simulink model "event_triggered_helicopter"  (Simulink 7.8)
settings: Solver=ode45  StartTime=0.0  StopTime=89  RelTol=1e-3
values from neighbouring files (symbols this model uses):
  d = lambda*0.5    [main_epsilon.m]    (also in main_rho_tau.m = 0.5)
undefined symbols (not defined in the file or in its folder): Ac_epsilon, Ac_rho, Ac_tau, c_epsilon, DiscIntNeverNeededParam, epsilon_0, Epsilon_disc, g, J_epsilon, Ka, Kb, Kc, L_epsilon, L_rho, L_tau, la, lh, lw, m, M, M_bf, Rho_disc, Tau_disc
libraries: commnoisgen2 x6, dspswit3 x2

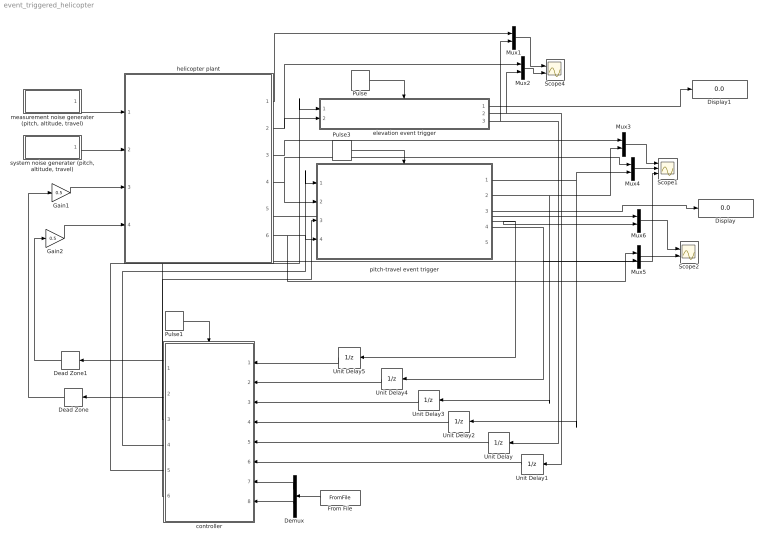
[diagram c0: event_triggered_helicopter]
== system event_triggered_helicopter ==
  Dead Zone : DeadZone  LowerValue=-1  UpperValue=1
  Dead Zone1 : DeadZone  LowerValue=-1  UpperValue=1
  Demux : Demux  Outputs=2
  Display : Display
  Display1 : Display
  From File : FromFile  FileName=input.mat  SampleTime=0
  Gain1 : Gain  Gain=0.5
  Gain2 : Gain  Gain=0.5
  Mux{1..6} (6 alike) : Mux  Inputs=2
  Pulse : DiscretePulseGenerator  PulseType=Time based  Period=0.005  PulseWidth=50
  Pulse1 : DiscretePulseGenerator  PulseType=Time based  Period=0.005  PulseWidth=30
  Pulse3 : DiscretePulseGenerator  PulseType=Time based  Period=0.005  PulseWidth=50
  Scope1 : Scope  NumInputPorts=3
  Scope2 : Scope  NumInputPorts=2
  Scope4 : Scope  NumInputPorts=2
  Unit Delay{,1..5} (6 alike) : UnitDelay  SampleTime=-1
  controller : Subsystem
  elevation event trigger : Subsystem
  helicopter plant : Subsystem
  "measurement noise generater (pitch, altitude, travel)" : Subsystem
  pitch-travel event trigger : Subsystem
  "system noise generater (pitch, altitude, travel)" : Subsystem
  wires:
  helicopter plant/2(altitude) -> elevation event trigger/2(elevation), Mux2/1
  Pulse/1 -> elevation event trigger/Trigger
  Mux1/1 -> Scope4/1
  Pulse1/1 -> controller/Trigger
  helicopter plant/5(travel rate) -> Mux6/1
  helicopter plant/3(pitch rate) -> Mux3/1
  controller/1(Vb) -> Dead Zone1/1
  Gain2/1 -> helicopter plant/4(Tb)
  controller/2(Vf) -> Dead Zone/1
  Gain1/1 -> helicopter plant/3(Tf)
  controller/5(u_elv) -> elevation event trigger/1(u_elv)
  From File/1 -> Demux/1
  Demux/2 -> controller/8(travel_rate_offset)
  Demux/1 -> controller/7(elevation_offset)
  helicopter plant/1(altitude rate) -> Mux1/1
  Mux2/1 -> Scope4/2
  elevation event trigger/3(remote estimated elevation rate) -> Unit Delay/1, Mux1/2
  elevation event trigger/2(remote estimated elevation) -> Unit Delay1/1, Mux2/2
  Unit Delay/1 -> controller/5(elevation_rate)
  Unit Delay1/1 -> controller/6(elevation)
  helicopter plant/4(pitch) -> pitch-travel event trigger/2(pitch), Mux4/1
  Unit Delay2/1 -> controller/4(pitch)
  Mux3/1 -> Scope1/1
  Mux4/1 -> Scope1/2
  Pulse3/1 -> pitch-travel event trigger/Trigger
  helicopter plant/6(travel) -> pitch-travel event trigger/4(travel), Mux5/1
  controller/3(u_trv) -> pitch-travel event trigger/3(u_trv)
  controller/4(u_pth) -> pitch-travel event trigger/1(u_pth)
  Mux5/1 -> Scope2/2
  pitch-travel event trigger/4("remote estimated travel ") -> Unit Delay4/1, Mux5/2
  Unit Delay3/1 -> controller/3(pitch_rate)
  Unit Delay4/1 -> controller/2(travel)
  pitch-travel event trigger/5(remote estimated travel rate) -> Mux6/2, Unit Delay5/1
  Mux6/1 -> Scope2/1
  Unit Delay5/1 -> controller/1(travel_rate)
  "measurement noise generater (pitch, altitude, travel)"/1(measurement noise) -> helicopter plant/1("measurement noise (pitch, altitude, travel)")
  "system noise generater (pitch, altitude, travel)"/1(system noise) -> helicopter plant/2("system noise (pitch, altitude, travel)")
  Dead Zone/1 -> Gain1/1
  Dead Zone1/1 -> Gain2/1
  pitch-travel event trigger/1(remote estimated pitch) -> Mux4/2, Unit Delay2/1
  pitch-travel event trigger/2(remote estimated pitch rate) -> Mux3/2, Unit Delay3/1
  pitch-travel event trigger/3(transmission times) -> Display/1
  elevation event trigger/1(elevation transmission times) -> Display1/1
  controller/6(pitch_offset) -> Scope1/3

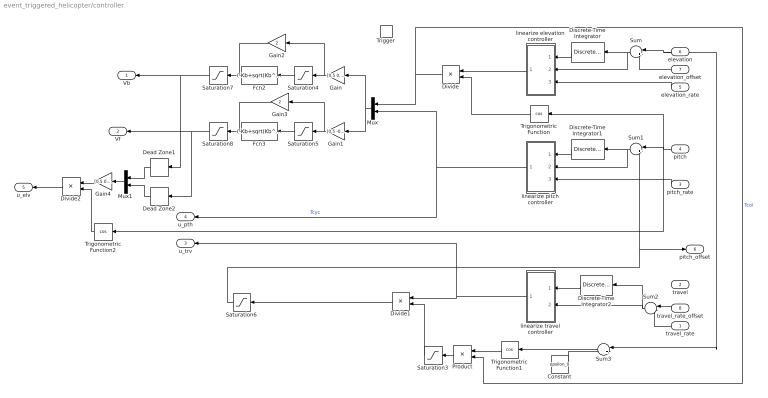
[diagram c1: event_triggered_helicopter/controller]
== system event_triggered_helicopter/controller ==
  travel_rate : Inport
  travel : Inport  Port=2
  pitch_rate : Inport  Port=3
  pitch : Inport  Port=4
  elevation_rate : Inport  Port=5
  elevation : Inport  Port=6
  elevation_offset : Inport  Port=7
  travel_rate_offset : Inport  Port=8
  Trigger : TriggerPort
  Constant : Constant  Value=epsilon_0
  Dead Zone1 : DeadZone  LowerValue=-1  UpperValue=1
  Dead Zone2 : DeadZone  LowerValue=-1  UpperValue=1
  Discrete-Time Integrator : DiscreteIntegrator  SampleTime=-1  LimitOutput=on  UpperSaturationLimit=1.8  LowerSaturationLimit=-1.8  ICPrevOutput=DiscIntNeverNeededParam  ICPrevScaledInput=DiscIntNeverNeededParam
  Discrete-Time Integrator1 : DiscreteIntegrator  SampleTime=-1  LimitOutput=on  UpperSaturationLimit=0.5  LowerSaturationLimit=-0.5  ICPrevOutput=DiscIntNeverNeededParam  ICPrevScaledInput=DiscIntNeverNeededParam
  Discrete-Time Integrator2 : DiscreteIntegrator  SampleTime=-1  LimitOutput=on  UpperSaturationLimit=0.12  LowerSaturationLimit=-0.12  ICPrevOutput=DiscIntNeverNeededParam  ICPrevScaledInput=DiscIntNeverNeededParam
  Divide : Product  Inputs=*/
  Divide1 : Product  Inputs=*/
  Divide2 : Product  Inputs=**
  Fcn2 : Fcn  Expr=(-Kb+sqrt(Kb^2-4*Ka*(Kc-u(1))))/(2*Ka)
  Fcn3 : Fcn  Expr=(-Kb+sqrt(Kb^2-4*Ka*(Kc-u(1))))/(2*Ka)
  Gain : Gain  Gain=[0.5 0.5]  Multiplication=Matrix(K*u)
  Gain1 : Gain  Gain=[0.5 -0.5]  Multiplication=Matrix(K*u)
  Gain2 : Gain  Gain=2
  Gain3 : Gain  Gain=2
  Gain4 : Gain  Gain=[0.5 0.5]  Multiplication=Matrix(K*u)
  Mux : Mux  Inputs=2
  Mux1 : Mux  Inputs=2
  Product : Product
  Saturation3 : Saturate  UpperLimit=inf  LowerLimit=0.8
  Saturation4 : Saturate  UpperLimit=1  LowerLimit=-0.0012
  Saturation5 : Saturate  UpperLimit=1  LowerLimit=-0.0012
  Saturation6 : Saturate  UpperLimit=0.6  LowerLimit=-0.6
  Saturation7 : Saturate  UpperLimit=4.99  LowerLimit=-4.99
  Saturation8 : Saturate  UpperLimit=4.99  LowerLimit=-4.99
  Sum : Sum  Inputs=|+-
  Sum1 : Sum  Inputs=|+-
  Sum2 : Sum  Inputs=|-+
  Sum3 : Sum  Inputs=|+-
  Trigonometric Function : Trigonometry  Operator=cos
  Trigonometric Function1 : Trigonometry  Operator=cos
  Trigonometric Function2 : Trigonometry  Operator=cos
  linearize elevation controller : Subsystem
  linearize pitch controller : Subsystem
  linearize travel controller : Subsystem
  Vb : Outport
  Vf : Outport  Port=2
  u_trv : Outport  Port=3
  u_pth : Outport  Port=4
  u_elv : Outport  Port=5
  pitch_offset : Outport  Port=6
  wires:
  elevation/1 -> Sum/1, Sum3/1
  elevation_offset/1 -> Sum/2
  Sum/1 -> linearize elevation controller/2(P), Discrete-Time Integrator/1
  Discrete-Time Integrator/1 -> linearize elevation controller/1(I)
  elevation_rate/1 -> linearize elevation controller/3(D)
  pitch/1 -> Sum1/1, Trigonometric Function2/1, Trigonometric Function/1
  Sum1/1 -> linearize pitch controller/2(P), Discrete-Time Integrator1/1
  pitch_rate/1 -> linearize pitch controller/3(D)
  travel_rate_offset/1 -> Sum2/1
  travel_rate/1 -> Sum2/2
  Sum2/1 -> Discrete-Time Integrator2/1, linearize travel controller/2(P)
  Discrete-Time Integrator2/1 -> linearize travel controller/1(I)
  Sum3/1 -> Trigonometric Function1/1
  Trigonometric Function1/1 -> Product/1
  Divide/1 -> Mux/1, Product/2  "Tcol"
  Product/1 -> Saturation3/1
  Saturation3/1 -> Divide1/2
  Mux/1 -> Gain/1, Gain1/1
  Gain/1 -> Saturation4/1, Gain2/1
  Gain1/1 -> Saturation5/1, Gain3/1
  Divide1/1 -> Saturation6/1
  Saturation7/1 -> Vb/1, Dead Zone1/1
  Saturation8/1 -> Vf/1, Dead Zone2/1
  Constant/1 -> Sum3/2
  Saturation4/1 -> Fcn2/1
  Saturation5/1 -> Fcn3/1
  Trigonometric Function/1 -> Divide/2
  Discrete-Time Integrator1/1 -> linearize pitch controller/1(I)
  Gain2/1 -> Saturation7/1
  Gain3/1 -> Saturation8/1
  linearize pitch controller/1(u_pth) -> Mux/2, u_pth/1  "Tcyc"
  linearize travel controller/1(u_trv) -> Divide1/1, u_trv/1
  linearize elevation controller/1(u_elv) -> Divide/1
  Dead Zone1/1 -> Mux1/1
  Dead Zone2/1 -> Mux1/2
  Mux1/1 -> Gain4/1
  Gain4/1 -> Divide2/1
  Trigonometric Function2/1 -> Divide2/2
  Divide2/1 -> u_elv/1
  Saturation6/1 -> Sum1/2, pitch_offset/1

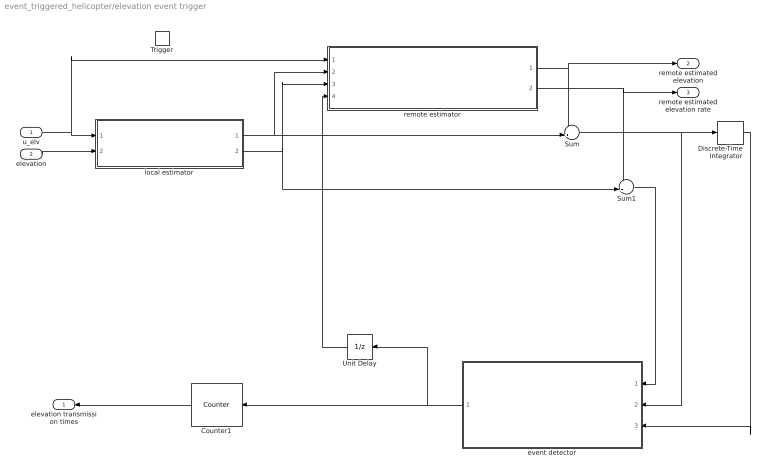
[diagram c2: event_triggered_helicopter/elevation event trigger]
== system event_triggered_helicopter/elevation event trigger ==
  u_elv : Inport
  elevation : Inport  Port=2
  Trigger : TriggerPort
  Counter1 : dspswit3/Counter  Direction=Up  CountEvent=Non-zero sample  CounterSize=User defined  MaxCount=20000  InitialCount=0  Output=Count  HitValue=32  ResetInput=off  SamplesPerFrame=1  Ts=1  CntDtype=int32  HitDtype=Logical
  Discrete-Time Integrator : DiscreteIntegrator  SampleTime=-1  ICPrevOutput=DiscIntNeverNeededParam  ICPrevScaledInput=DiscIntNeverNeededParam
  Sum : Sum  Inputs=-+|
  Sum1 : Sum  Inputs=-+|
  Unit Delay : UnitDelay  SampleTime=-1
  event detector : Subsystem
  local estimator : Subsystem
  remote estimator : Subsystem
  elevation transmission times : Outport
  remote estimated elevation : Outport  Port=2
  remote estimated elevation rate : Outport  Port=3
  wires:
  u_elv/1 -> local estimator/1(u_elv), remote estimator/1(u_elv)
  elevation/1 -> local estimator/2(elevation)
  local estimator/1(local estimated elevation) -> remote estimator/2("local estimated elevation "), Sum/2
  remote estimator/1(remote estimated elevation) -> remote estimated elevation/1, Sum/1
  local estimator/2(local estimated elevation rate) -> remote estimator/3(local estimated elevation rate), Sum1/2
  Counter1/1 -> elevation transmission times/1
  Unit Delay/1 -> remote estimator/4(transmit signal)
  remote estimator/2(remote estimated elevation rate) -> remote estimated elevation rate/1, Sum1/1
  event detector/1(transmit signal) -> Unit Delay/1, Counter1/1
  Sum/1 -> Discrete-Time Integrator/1, event detector/2(elevation_p)
  Sum1/1 -> event detector/1(elevation_d)
  Discrete-Time Integrator/1 -> event detector/3(elevation_i)

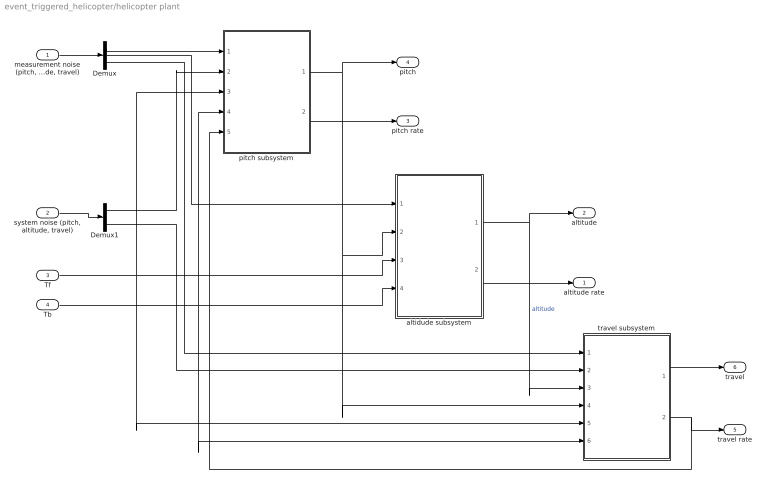
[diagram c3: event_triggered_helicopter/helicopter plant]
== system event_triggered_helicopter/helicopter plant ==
  "measurement noise (pitch, altitude, travel)" : Inport
  "system noise (pitch, altitude, travel)" : Inport  Port=2
  Tf : Inport  Port=3
  Tb : Inport  Port=4
  Demux : Demux  Outputs=3
  Demux1 : Demux  Outputs=3
  altidude subsystem : Subsystem
  pitch subsystem : Subsystem
  travel subsystem : Subsystem
  altitude rate : Outport
  altitude : Outport  Port=2
  pitch rate : Outport  Port=3
  pitch : Outport  Port=4
  travel rate : Outport  Port=5
  travel : Outport  Port=6
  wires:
  pitch subsystem/1(pitch) -> pitch/1, altidude subsystem/2(pitch), travel subsystem/4(pitch)
  altidude subsystem/1(altitude) -> altitude/1, travel subsystem/3(altitude)  "altitude"
  pitch subsystem/2(pitch rate) -> pitch rate/1
  altidude subsystem/2(altitude rate) -> altitude rate/1
  travel subsystem/1(travel) -> travel/1
  travel subsystem/2(travel rate) -> pitch subsystem/5(travel_rate), travel rate/1
  Demux/1 -> pitch subsystem/1(measurement noise)
  Demux/2 -> altidude subsystem/1(measurement noise)
  Demux/3 -> travel subsystem/1(measurement noise)
  "measurement noise (pitch, altitude, travel)"/1 -> Demux/1
  Demux1/1 -> pitch subsystem/2(system noise)
  Demux1/3 -> travel subsystem/2(system noise)
  Tf/1 -> altidude subsystem/3(Tf), travel subsystem/5(Tf), pitch subsystem/3(Tf)
  Tb/1 -> altidude subsystem/4(Tb), pitch subsystem/4(Tb), travel subsystem/6(Tb)
  "system noise (pitch, altitude, travel)"/1 -> Demux1/1

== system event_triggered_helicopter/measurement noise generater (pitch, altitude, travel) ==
  Mux : Mux  Inputs=3
  altitude Noise Generator : commnoisgen2/Gaussian Noise Generator  m=0  d=1.857e-8  s=41  Ts=0.0025  frameBased=off  sampPerFrame=1  orient=off  outDataType=double
  pitch noise Generator : commnoisgen2/Gaussian Noise Generator  m=0  d=1.857e-8  s=1  Ts=0.0025  frameBased=off  sampPerFrame=1  orient=off  outDataType=double
  travel noise Generator : commnoisgen2/Gaussian Noise Generator  m=0  d=1.857e-8  s=3  Ts=0.0025  frameBased=off  sampPerFrame=1  orient=off  outDataType=double
  measurement noise : Outport
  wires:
  pitch noise Generator/1 -> Mux/1
  altitude Noise Generator/1 -> Mux/2
  travel noise Generator/1 -> Mux/3
  Mux/1 -> measurement noise/1

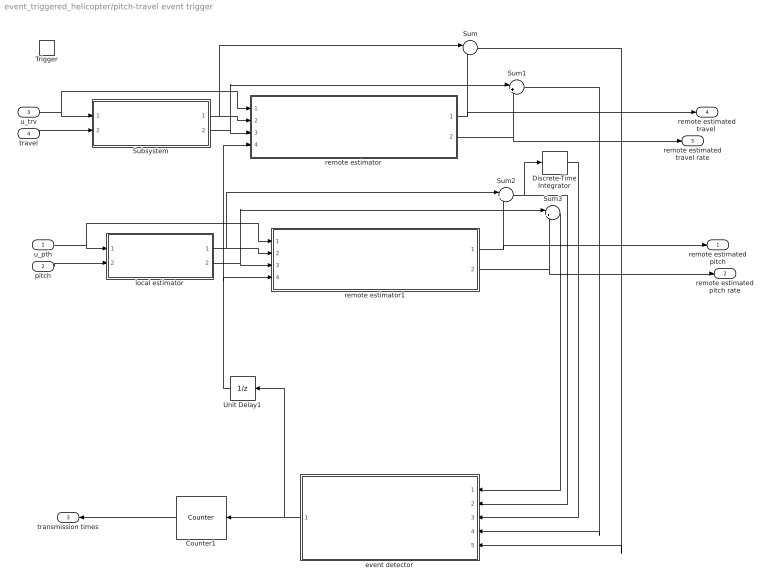
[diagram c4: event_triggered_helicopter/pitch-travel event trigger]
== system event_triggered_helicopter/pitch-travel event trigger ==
  u_pth : Inport
  pitch : Inport  Port=2
  u_trv : Inport  Port=3
  travel : Inport  Port=4
  Trigger : TriggerPort
  Counter1 : dspswit3/Counter  Direction=Up  CountEvent=Non-zero sample  CounterSize=User defined  MaxCount=20000  InitialCount=0  Output=Count  HitValue=32  ResetInput=off  SamplesPerFrame=1  Ts=1  CntDtype=int32  HitDtype=Logical
  Discrete-Time Integrator : DiscreteIntegrator  SampleTime=-1  ICPrevOutput=DiscIntNeverNeededParam  ICPrevScaledInput=DiscIntNeverNeededParam
  Subsystem : Subsystem
  Sum{,1..3} (4 alike) : Sum  Inputs=|+-
  Unit Delay1 : UnitDelay  SampleTime=-1
  event detector : Subsystem
  local estimator : Subsystem
  remote estimator : Subsystem
  remote estimator1 : Subsystem
  remote estimated pitch : Outport
  remote estimated pitch rate : Outport  Port=2
  transmission times : Outport  Port=3
  "remote estimated travel " : Outport  Port=4
  remote estimated travel rate : Outport  Port=5
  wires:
  u_trv/1 -> Subsystem/1(u_trv), remote estimator/1(u_trv)
  travel/1 -> Subsystem/2(travel)
  Subsystem/2(local estimated travel rate) -> remote estimator/3(local estimated travel rate), Sum1/1
  remote estimator/2(remote estimated travel rate) -> remote estimated travel rate/1, Sum1/2
  remote estimator/1(remote estimated travel) -> "remote estimated travel "/1, Sum/2
  Subsystem/1(local estimated travel) -> remote estimator/2(local estimated travel), Sum/1
  Counter1/1 -> transmission times/1
  event detector/1(transmit signal) -> Unit Delay1/1, Counter1/1
  u_pth/1 -> local estimator/1(u_pth), remote estimator1/1(u_pth)
  pitch/1 -> local estimator/2(pitch)
  local estimator/1(local estimated pitch) -> remote estimator1/2(local estimated pitch), Sum2/1
  local estimator/2(local estimated pitch rate) -> remote estimator1/3(local estimated pitch rate), Sum3/1
  remote estimator1/1(remote estimated pitch) -> remote estimated pitch/1, Sum2/2
  remote estimator1/2(remote estimated pitch rate) -> remote estimated pitch rate/1, Sum3/2
  Sum2/1 -> Discrete-Time Integrator/1, event detector/2(pitch_p)
  Sum3/1 -> event detector/1(pitch_d)
  Discrete-Time Integrator/1 -> event detector/3(pitch_i)
  Sum1/1 -> event detector/4(travel_d)
  Sum/1 -> event detector/5(travel_p)
  Unit Delay1/1 -> remote estimator/4(transmit signal), remote estimator1/4(transmit signal)

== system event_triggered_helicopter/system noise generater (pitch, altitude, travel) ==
  Mux : Mux  Inputs=3
  altitude Noise Generator : commnoisgen2/Gaussian Noise Generator  m=0  d=1e-12  s=7  Ts=0.0025  frameBased=off  sampPerFrame=1  orient=off  outDataType=double
  pitch noise Generator : commnoisgen2/Gaussian Noise Generator  m=0  d=1e-12  s=5  Ts=0.0025  frameBased=off  sampPerFrame=1  orient=off  outDataType=double
  travel Noise Generator : commnoisgen2/Gaussian Noise Generator  m=0  d=1e-12  s=11  Ts=0.0025  frameBased=off  sampPerFrame=1  orient=off  outDataType=double
  system noise : Outport
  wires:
  pitch noise Generator/1 -> Mux/1
  altitude Noise Generator/1 -> Mux/2
  Mux/1 -> system noise/1
  travel Noise Generator/1 -> Mux/3

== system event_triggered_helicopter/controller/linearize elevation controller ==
  I : Inport
  P : Inport  Port=2
  D : Inport  Port=3
  Gain : Gain  Gain=[-7 -44 -68]  Multiplication=Matrix(K*u)
  Mux : Mux  Inputs=3
  u_elv : Outport
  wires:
  Mux/1 -> Gain/1
  I/1 -> Mux/1
  Gain/1 -> u_elv/1
  P/1 -> Mux/2
  D/1 -> Mux/3

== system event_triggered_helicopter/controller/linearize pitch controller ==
  I : Inport
  P : Inport  Port=2
  D : Inport  Port=3
  Gain : Gain  Gain=[-3.5 -30 -20]  Multiplication=Matrix(K*u)
  Mux : Mux  Inputs=3
  u_pth : Outport
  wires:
  Mux/1 -> Gain/1
  I/1 -> Mux/1
  Gain/1 -> u_pth/1
  P/1 -> Mux/2
  D/1 -> Mux/3

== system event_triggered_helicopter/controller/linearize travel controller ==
  I : Inport
  P : Inport  Port=2
  Gain : Gain  Gain=[3.5 20]  Multiplication=Matrix(K*u)
  Mux : Mux  Inputs=2
  u_trv : Outport
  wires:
  Mux/1 -> Gain/1
  I/1 -> Mux/1
  Gain/1 -> u_trv/1
  P/1 -> Mux/2

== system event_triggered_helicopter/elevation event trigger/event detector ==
  elevation_d : Inport
  elevation_p : Inport  Port=2
  elevation_i : Inport  Port=3
  Constant : Constant
  Constant1 : Constant  Value=0
  Fcn : Fcn  Expr=|
      | 7.5776*u(1)^6 + 0.064983*u(1)^5*u(2) + 0.0017543*u(1)^5*u(3) - 3.0262*u(1)^4*u(2)^2 
      |   - 0.0045238*u(1)^4*u(2)*u(3) + 3.6614*u(1)^4*u(3)^2 - 4.7737*u(1)^4 - 0.023298
      |   *u(1)^3*u(2)^3 - 0.001249*u(1)^3*u(2)^2*u(3) - 0.010189*u(1)^3*u(2)*u(3)^2 - 0.32359
      |   *u(1)^3*u(2) + 0.00012009*u(1)^3*u(3)^3 - 0.0078634*u(1)^3*u(3) + 1.106*u(1)^2*u(2)^4 
      |   + 0.0035527*u(1)^2*u(2)^3*u(3) - 0.99402*u(1)^2*u(2)^2*u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
  Mux : Mux  Inputs=3
  Switch : Switch
  transmit signal : Outport
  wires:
  elevation_d/1 -> Mux/3
  elevation_p/1 -> Mux/2
  elevation_i/1 -> Mux/1
  Mux/1 -> Fcn/1
  Fcn/1 -> Switch/2
  Constant/1 -> Switch/1
  Constant1/1 -> Switch/3
  Switch/1 -> transmit signal/1

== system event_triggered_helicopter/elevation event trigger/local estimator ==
  u_elv : Inport
  elevation : Inport  Port=2
  Demux : Demux  Outputs=2
  Gain2 : Gain  Gain=[Ac_epsilon(2:3,2:3) Epsilon_disc.B(2:3) L_epsilon(2:3,2)]  Multiplication=Matrix(K*u)
  Mux : Mux  Inputs=3
  Unit Delay : UnitDelay  SampleTime=-1
  local estimated elevation : Outport
  local estimated elevation rate : Outport  Port=2
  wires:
  Unit Delay/1 -> Mux/1
  u_elv/1 -> Mux/2
  elevation/1 -> Mux/3
  Mux/1 -> Gain2/1
  Gain2/1 -> Demux/1, Unit Delay/1
  Demux/1 -> local estimated elevation/1
  Demux/2 -> local estimated elevation rate/1

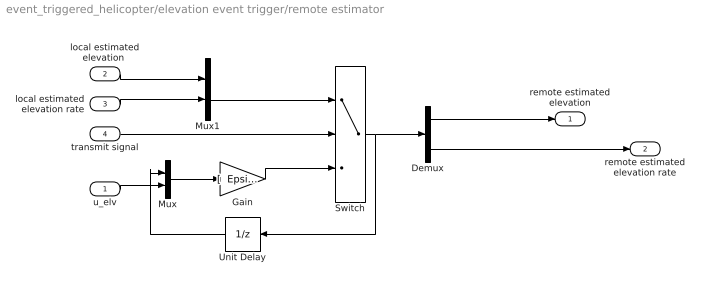
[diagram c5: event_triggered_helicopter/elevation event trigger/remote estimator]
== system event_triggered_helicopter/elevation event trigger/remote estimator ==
  u_elv : Inport
  "local estimated elevation " : Inport  Port=2
  local estimated elevation rate : Inport  Port=3
  transmit signal : Inport  Port=4
  Demux : Demux  Outputs=2
  Gain : Gain  Gain="[  Epsilon_disc.A(2:3,2:3)  Epsilon_disc.B(2:3)]"  Multiplication=Matrix(K*u)
  Mux : Mux  Inputs=2
  Mux1 : Mux  Inputs=2
  Switch : Switch  Threshold=1
  Unit Delay : UnitDelay  SampleTime=-1
  remote estimated elevation : Outport
  remote estimated elevation rate : Outport  Port=2
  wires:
  Mux/1 -> Gain/1
  u_elv/1 -> Mux/2
  Demux/1 -> remote estimated elevation/1
  Demux/2 -> remote estimated elevation rate/1
  Gain/1 -> Switch/3
  transmit signal/1 -> Switch/2
  Switch/1 -> Demux/1, Unit Delay/1
  Unit Delay/1 -> Mux/1
  "local estimated elevation "/1 -> Mux1/1
  local estimated elevation rate/1 -> Mux1/2
  Mux1/1 -> Switch/1

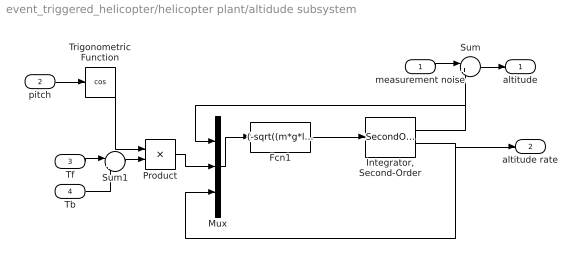
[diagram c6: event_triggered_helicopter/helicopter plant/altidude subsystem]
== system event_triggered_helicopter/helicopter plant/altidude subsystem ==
  measurement noise : Inport
  pitch : Inport  Port=2
  Tf : Inport  Port=3
  Tb : Inport  Port=4
  Fcn1 : Fcn  Expr=(-sqrt((m*g*lw-M*g*la)^2+((m+M)*g*d)^2)*sin(u(1))+(la+d*tan(u(1)+epsilon_0))*u(2)-c_epsilon*u(3))/J_epsilon
  "Integrator, Second-Order" : SecondOrderIntegrator
  Mux : Mux  Inputs=3
  Product : Product
  Sum : Sum  Inputs=|++
  Sum1 : Sum  Inputs=|++
  Trigonometric Function : Trigonometry  Operator=cos
  altitude : Outport
  altitude rate : Outport  Port=2
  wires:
  Fcn1/1 -> "Integrator, Second-Order"/1
  "Integrator, Second-Order"/1 -> Sum/2, Mux/1
  measurement noise/1 -> Sum/1
  Sum/1 -> altitude/1
  "Integrator, Second-Order"/2 -> altitude rate/1, Mux/3
  Tf/1 -> Sum1/1
  Tb/1 -> Sum1/2
  Mux/1 -> Fcn1/1
  Sum1/1 -> Product/2
  pitch/1 -> Trigonometric Function/1
  Product/1 -> Mux/2
  Trigonometric Function/1 -> Product/1

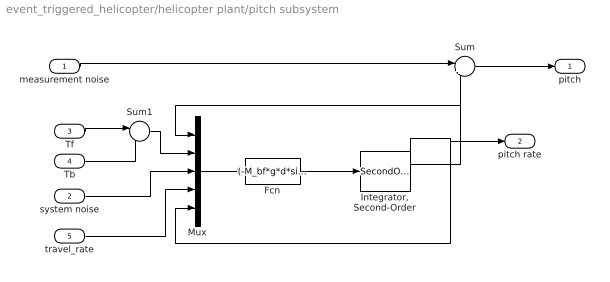
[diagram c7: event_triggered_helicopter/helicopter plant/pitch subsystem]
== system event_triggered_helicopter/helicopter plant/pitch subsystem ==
  measurement noise : Inport
  system noise : Inport  Port=2
  Tf : Inport  Port=3
  Tb : Inport  Port=4
  travel_rate : Inport  Port=5
  Fcn : Fcn  Expr=(-M_bf*g*d*sin(u(1))+lh*u(2)-0.003*u(5)+0.003*u(4)+u(3))/(0.01)
  "Integrator, Second-Order" : SecondOrderIntegrator
  Mux : Mux  Inputs=5
  Sum : Sum  Inputs=|++
  Sum1 : Sum  Inputs=|-+
  pitch : Outport
  pitch rate : Outport  Port=2
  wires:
  Mux/1 -> Fcn/1
  Fcn/1 -> "Integrator, Second-Order"/1
  "Integrator, Second-Order"/1 -> Sum/2, Mux/1
  measurement noise/1 -> Sum/1
  Sum/1 -> pitch/1
  "Integrator, Second-Order"/2 -> pitch rate/1, Mux/5
  system noise/1 -> Mux/3
  Tf/1 -> Sum1/1
  Tb/1 -> Sum1/2
  travel_rate/1 -> Mux/4
  Sum1/1 -> Mux/2

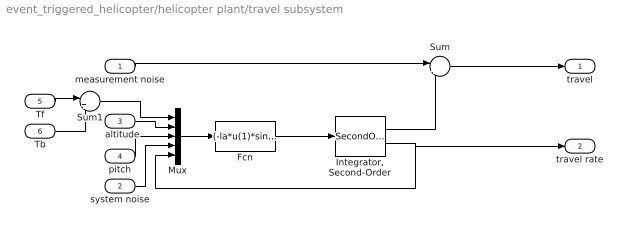
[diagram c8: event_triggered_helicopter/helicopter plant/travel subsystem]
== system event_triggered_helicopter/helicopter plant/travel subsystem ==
  measurement noise : Inport
  system noise : Inport  Port=2
  altitude : Inport  Port=3
  pitch : Inport  Port=4
  Tf : Inport  Port=5
  Tb : Inport  Port=6
  Fcn : Fcn  Expr=(-la*u(1)*sin(u(3))*cos(u(2)+epsilon_0)-0.25*u(5)+u(4))/4
  "Integrator, Second-Order" : SecondOrderIntegrator
  Mux : Mux  Inputs=5
  Sum : Sum  Inputs=|++
  Sum1 : Sum  Inputs=|++
  travel : Outport
  travel rate : Outport  Port=2
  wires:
  Mux/1 -> Fcn/1
  "Integrator, Second-Order"/1 -> Sum/2
  measurement noise/1 -> Sum/1
  Sum/1 -> travel/1
  altitude/1 -> Mux/2
  "Integrator, Second-Order"/2 -> travel rate/1, Mux/5
  Sum1/1 -> Mux/1
  pitch/1 -> Mux/3
  system noise/1 -> Mux/4
  Tf/1 -> Sum1/1
  Tb/1 -> Sum1/2
  Fcn/1 -> "Integrator, Second-Order"/1

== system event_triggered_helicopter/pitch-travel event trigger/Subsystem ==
  u_trv : Inport
  travel : Inport  Port=2
  Demux : Demux  Outputs=2
  Gain2 : Gain  Gain=[Ac_tau Tau_disc.B L_tau]  Multiplication=Matrix(K*u)
  Mux : Mux  Inputs=3
  Unit Delay : UnitDelay  SampleTime=-1
  local estimated travel : Outport
  local estimated travel rate : Outport  Port=2
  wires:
  Gain2/1 -> Unit Delay/1, Demux/1
  Unit Delay/1 -> Mux/1
  Mux/1 -> Gain2/1
  u_trv/1 -> Mux/2
  travel/1 -> Mux/3
  Demux/1 -> local estimated travel/1
  Demux/2 -> local estimated travel rate/1

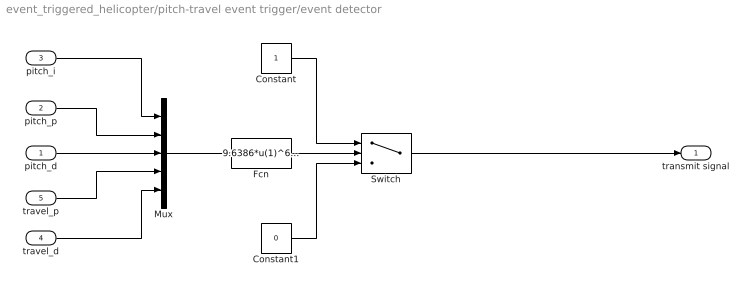
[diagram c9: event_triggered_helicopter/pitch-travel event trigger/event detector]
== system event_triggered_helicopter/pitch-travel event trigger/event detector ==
  pitch_d : Inport
  pitch_p : Inport  Port=2
  pitch_i : Inport  Port=3
  travel_d : Inport  Port=4
  travel_p : Inport  Port=5
  Constant : Constant
  Constant1 : Constant  Value=0
  Fcn : Fcn  Expr=|
      | 9.6386*u(1)^6 + 0.12666*u(1)^5*u(2) + 0.042053*u(1)^5*u(3) - 2.5554*u(1)^4*u(2)^2 + 0.33103
      |   *u(1)^4*u(2)*u(3) + 7.9379*u(1)^4*u(3)^2 - 10.9657*u(1)^4 - 0.064688*u(1)^3*u(2)^3 - 0.021023
      |   *u(1)^3*u(2)^2*u(3) + 0.024183*u(1)^3*u(2)*u(3)^2 - 0.22301*u(1)^3*u(2) + 0.0071206*u(1)^3
      |   *u(3)^3 - 0.031978*u(1)^3*u(3) + 2.0293*u(1)^2*u(2)^4 - 0.25656*u(1)^2*u(2)^3*u(3) - 1.2305
      |   *u(1)^2*u(2)^2*u(3)^2 +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
  Mux : Mux  Inputs=5
  Switch : Switch
  transmit signal : Outport
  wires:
  pitch_d/1 -> Mux/3
  pitch_p/1 -> Mux/2
  pitch_i/1 -> Mux/1
  travel_p/1 -> Mux/4
  travel_d/1 -> Mux/5
  Mux/1 -> Fcn/1
  Fcn/1 -> Switch/2
  Constant/1 -> Switch/1
  Constant1/1 -> Switch/3
  Switch/1 -> transmit signal/1

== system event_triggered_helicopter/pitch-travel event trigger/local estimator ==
  u_pth : Inport
  pitch : Inport  Port=2
  Demux : Demux  Outputs=2
  Gain2 : Gain  Gain=[Ac_rho(2:3,2:3) Rho_disc.B(2:3) L_rho(2:3,2)]  Multiplication=Matrix(K*u)
  Mux : Mux  Inputs=3
  Unit Delay : UnitDelay  SampleTime=-1
  local estimated pitch : Outport
  local estimated pitch rate : Outport  Port=2
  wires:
  Gain2/1 -> Unit Delay/1, Demux/1
  Unit Delay/1 -> Mux/1
  Mux/1 -> Gain2/1
  u_pth/1 -> Mux/2
  pitch/1 -> Mux/3
  Demux/1 -> local estimated pitch/1
  Demux/2 -> local estimated pitch rate/1

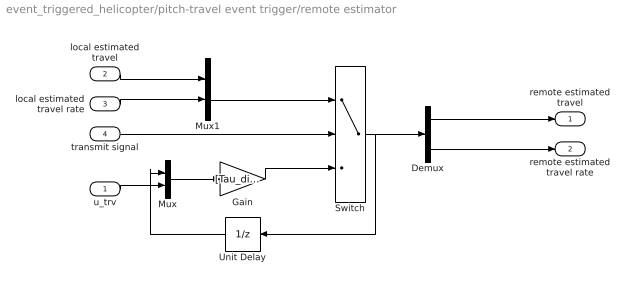
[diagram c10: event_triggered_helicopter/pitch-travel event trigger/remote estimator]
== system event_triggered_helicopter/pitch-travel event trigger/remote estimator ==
  u_trv : Inport
  local estimated travel : Inport  Port=2
  local estimated travel rate : Inport  Port=3
  transmit signal : Inport  Port=4
  Demux : Demux  Outputs=2
  Gain : Gain  Gain=[Tau_disc.A Tau_disc.B]  Multiplication=Matrix(K*u)
  Mux : Mux  Inputs=2
  Mux1 : Mux  Inputs=2
  Switch : Switch  Threshold=0.5
  Unit Delay : UnitDelay  SampleTime=-1
  remote estimated travel : Outport
  remote estimated travel rate : Outport  Port=2
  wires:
  Mux/1 -> Gain/1
  u_trv/1 -> Mux/2
  Demux/1 -> remote estimated travel/1
  Demux/2 -> remote estimated travel rate/1
  Gain/1 -> Switch/3
  transmit signal/1 -> Switch/2
  Switch/1 -> Unit Delay/1, Demux/1
  Unit Delay/1 -> Mux/1
  local estimated travel/1 -> Mux1/1
  local estimated travel rate/1 -> Mux1/2
  Mux1/1 -> Switch/1

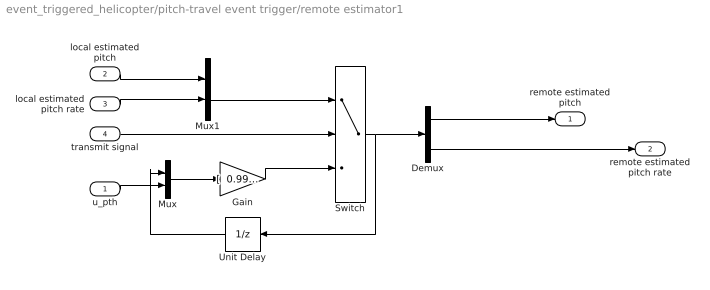
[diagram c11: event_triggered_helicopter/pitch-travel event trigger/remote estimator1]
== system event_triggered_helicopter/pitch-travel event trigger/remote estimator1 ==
  u_pth : Inport
  local estimated pitch : Inport  Port=2
  local estimated pitch rate : Inport  Port=3
  transmit signal : Inport  Port=4
  Demux : Demux  Outputs=2
  Gain : Gain  Gain=|  Multiplication=Matrix(K*u)
      | [  0.9999    0.0050    0.0002
      | ;   -0.0568    0.9984    0.0884]
  Mux : Mux  Inputs=2
  Mux1 : Mux  Inputs=2
  Switch : Switch  Threshold=.5
  Unit Delay : UnitDelay  SampleTime=-1
  remote estimated pitch : Outport
  remote estimated pitch rate : Outport  Port=2
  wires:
  Mux/1 -> Gain/1
  u_pth/1 -> Mux/2
  Demux/1 -> remote estimated pitch/1
  Demux/2 -> remote estimated pitch rate/1
  Gain/1 -> Switch/3
  transmit signal/1 -> Switch/2
  Switch/1 -> Unit Delay/1, Demux/1
  Unit Delay/1 -> Mux/1
  local estimated pitch/1 -> Mux1/1
  local estimated pitch rate/1 -> Mux1/2
  Mux1/1 -> Switch/1
